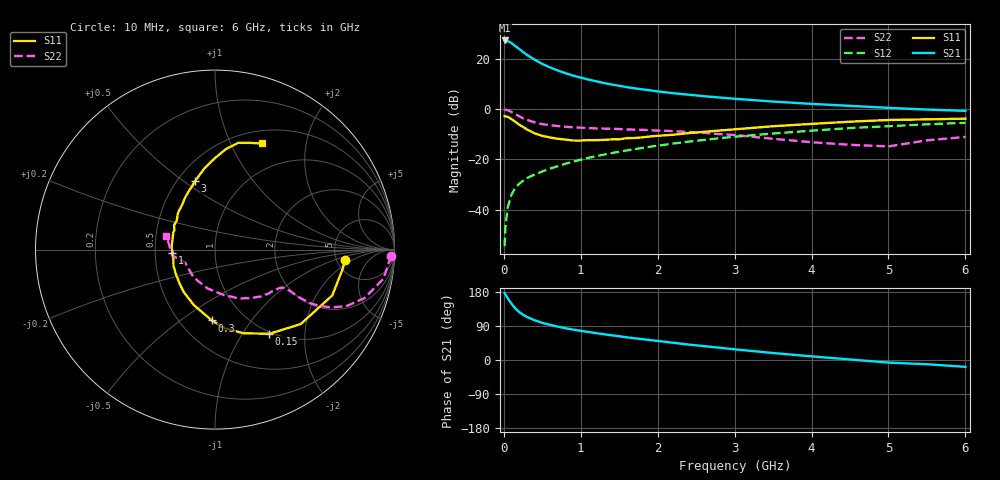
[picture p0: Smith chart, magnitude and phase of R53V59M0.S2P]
! SIEMENS Small Signal Semiconductors
! BFR183
! Si NPN RF Bipolar Junction Transistor in SOT23
! VCE = 3.5 V  IC = 9 mA
! Common Emitter S-Parameters:  May  1996
# GHz  S  MA  R  50
!  f  S11  S21  S12  S22
! GHz  MAG  ANG  MAG  ANG  MAG  ANG  MAG  ANG
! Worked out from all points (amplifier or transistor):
!   36 points, 10 MHz to 6 GHz, reference 50 ohm
!   highest |S21| = 27.3 dB at 10 MHz (marker M1)
!   |S21| within 3 dB of that: start of sweep to 183.8 MHz
!   unconditionally stable (mu >= 1): 814.1 MHz to 2.516 GHz
!   at 250 MHz: K = 0.59, MSG = 25.6 dB, |S12| = -28.5 dB
!   at 1.4 GHz: K = 1.05, MAG = 12.2 dB, |S12| = -17.5 dB
!   at 6 GHz: K = 0.89, MSG = 2.4 dB, |S12| = -5.4 dB
!   S11 on the Smith chart (normalised r, x): 10 MHz: 5.93, -1.43; 150 MHz: 0.97, -1.33; 300 MHz: 0.71, -0.66; 1 GHz: 0.62, -0.02; 3 GHz: 0.61, +0.55; 6 GHz: 0.65, +1.32
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0.01  0.7254 -4.5  23.08 176.6  0.0019 91.1  0.9811 -2.0
0.02  0.7198 -8.5  22.83 172.9  0.0045 84.2  0.9726 -4.0
0.05  0.7016 -21.3  22.5 163.1  0.0111 81.0  0.9523 -9.8
0.1  0.6327 -41.0  20.44 148.4  0.0201 73.5  0.8764 -17.9
0.15  0.5579 -57.2  17.87 135.8  0.0277 66.5  0.7958 -23.4
0.2  0.492 -71.3  15.65 126.5  0.0329 64.0  0.7191 -26.6
0.25  0.4417 -82.9  13.6 119.3  0.0378 61.9  0.6567 -28.4
0.3  0.395 -92.7  11.96 113.5  0.0426 61.7  0.6121 -29.3
0.4  0.3307 -110.8  9.595 105.0  0.0504 61.4  0.5456 -29.6
0.5  0.295 -125.8  7.891 98.0  0.0578 62.8  0.5028 -29.2
0.6  0.2729 -136.5  6.725 92.8  0.0658 63.3  0.4775 -28.9
0.7  0.2575 -147.7  5.861 88.1  0.0737 63.9  0.4608 -28.9
0.8  0.2483 -158.7  5.168 84.0  0.0822 63.9  0.4461 -29.1
1  0.2374 -176.0  4.215 77.0  0.0988 64.8  0.4277 -29.7
1.1  0.2424 177.0  3.869 73.9  0.1079 64.6  0.4208 -30.6
1.6  0.2659 149.0  2.729 59.8  0.1512 62.5  0.3952 -36.0
2.2  0.3093 126.2  2.071 45.5  0.2068 58.0  0.3661 -45.5
3  0.3965 106.4  1.607 28.2  0.2828 49.9  0.3059 -63.2
3.5  0.4573 97.3  1.412 18.4  0.3274 43.8  0.2578 -79.0
4.5  0.5626 83.9  1.161 1.4  0.4209 31.6  0.1955 -127.9
5.5  0.6263 71.7  0.98 -11.2  0.499 19.6  0.2399 -172.1
6  0.6462 66.2  0.923 -18.0  0.5356 11.8  0.2805 164.5
